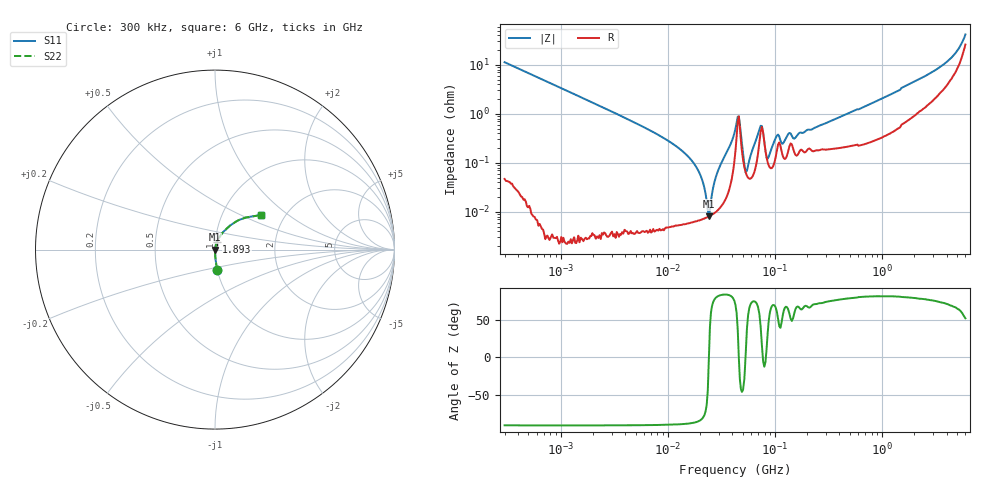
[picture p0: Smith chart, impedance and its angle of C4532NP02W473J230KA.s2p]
! S-Parameter Data Generated by TDK Corporation
! Copyright(C) 2024 TDK Corporation.
! All Rights Reserved.
! TDK P/N: C4532NP02W473J230KA (Multilayer Ceramic Chip Capacitor)
! Property: C=47nF
! Size(LxWxT): 4.5x3.2x2.3mm
! Model Type: s2p (Touchstone File Format Version 1.0)
! Frequency: DC=Yes Start=0.3MHz Stop=6000MHz 402points Log-sweep
! Model Generated on May 28, 2024
! Terms and conditions regarding TDK Simulation Models:
! 1)This simulation model is being provided solely for informational
!  purposes. Please refer to the specifications of the products in
!  terms of detailed characteristics of such products.
! 2)In no event shall TDK Corporation of any of its subsidiaries be
!  liable for any loss or damage arising, directly or indirectly,
!  from any information contained in this simulation model, including,
!  but not limited to loss or damages arising from any inaccuracies,
!  omissions or errors in connection with such information.
! 3)Any and all copyrights on this simulation model are owned by
!  TDK Corporation.  Duplication or redistribution of this simulation
!  model without prior written permission from TDK Corporation
!  is prohibited.
! 4)This simulation model is subject to any modification or change
!  without any prior notice.
! 5)Neither TDK Corporation nor any of its subsidiaries shall make any
!  warranty, express or implied, including but not limited to the
!  correctness, implied warranties of merchantability and fitness for
!  a particular purpose with respect to this simulation models.
! 6)The use of this simulation model shall be deemed to have consented
!  to the terms and conditions hereof.
! Port Assignments:
!  1 ---| |--- 2
! Applicable Conditions:
!  Temperature = 25 degC
!  DC Bias Voltage = 0 V
!  Small Signal Operation
# Hz S MA R 50
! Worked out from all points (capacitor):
!   401 points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, 300 kHz to 6 GHz, reference 50 ohm
!   read as one part in series: C = 47 nF near 317.3 kHz
!   lowest |Z| = 8.07 mohm at 24.2 MHz (marker M1)
!   series resonance near 24.22 MHz, so ESL is about 920 pH
!   S11 on the Smith chart (normalised r, x): 300 kHz: 1.00, -0.23; 1.893 GHz: 1.02, +0.08; 6 GHz: 1.52, +0.65
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300000  0.112 -83.3  0.9932 6.4  0.9932 6.4  0.112 -83.3
1586297  0.02123 -88.7  0.9997 1.2  0.9997 1.2  0.02123 -88.7
8158352  0.00371 -89.2  1 0.2  1 0.2  0.00371 -89.2
1.753708e7  0.0009712 -86.3  0.9999 0.1  0.9999 0.1  0.0009712 -86.3
2.087273e7  0.0004583 -81.2  0.9999 0.0  0.9999 0.0  0.0004583 -81.2
2.419584e7  8.07e-05 -2.1  0.9999 0.0  0.9999 0.0  8.07e-05 -2.1
2.879802e7  0.0006014 80.0  0.9999 -0.0  0.9999 -0.0  0.0006014 80.0
4.28954e7  0.004995 68.8  0.9982 -0.3  0.9982 -0.3  0.004995 68.8
4.605827e7  0.00881 -0.5  0.9912 0.0  0.9912 0.0  0.00881 -0.5
5.190961e7  0.0009128 -28.1  0.9992 0.0  0.9992 0.0  0.0009128 -28.1
5.481881e7  0.0006863 37.7  0.9995 -0.0  0.9995 -0.0  0.0006863 37.7
7.36264e7  0.005662 40.6  0.9957 -0.2  0.9957 -0.2  0.005662 40.6
8.566785e7  0.001211 32.6  0.999 -0.0  0.999 -0.0  0.001211 32.6
1.04351e8  0.003578 60.1  0.9982 -0.2  0.9982 -0.2  0.003578 60.1
1.181956e8  0.002444 54.9  0.9986 -0.1  0.9986 -0.1  0.002444 54.9
1.325118e8  0.003789 63.8  0.9983 -0.2  0.9983 -0.2  0.003789 63.8
1.554335e8  0.003242 63.2  0.9985 -0.2  0.9985 -0.2  0.003242 63.2
2.249926e8  0.004881 69.1  0.9983 -0.3  0.9983 -0.3  0.004881 69.1
1.174439e9  0.02413 79.4  0.9958 -1.4  0.9958 -1.4  0.02413 79.4
1.89308e9  0.04217 76.4  0.9909 -2.4  0.9909 -2.4  0.04217 76.4
3.976189e9  0.1076 65.0  0.9596 -5.8  0.9596 -5.8  0.1076 65.0
6e9  0.3198 37.1  0.7694 -14.5  0.7694 -14.5  0.3198 37.1
